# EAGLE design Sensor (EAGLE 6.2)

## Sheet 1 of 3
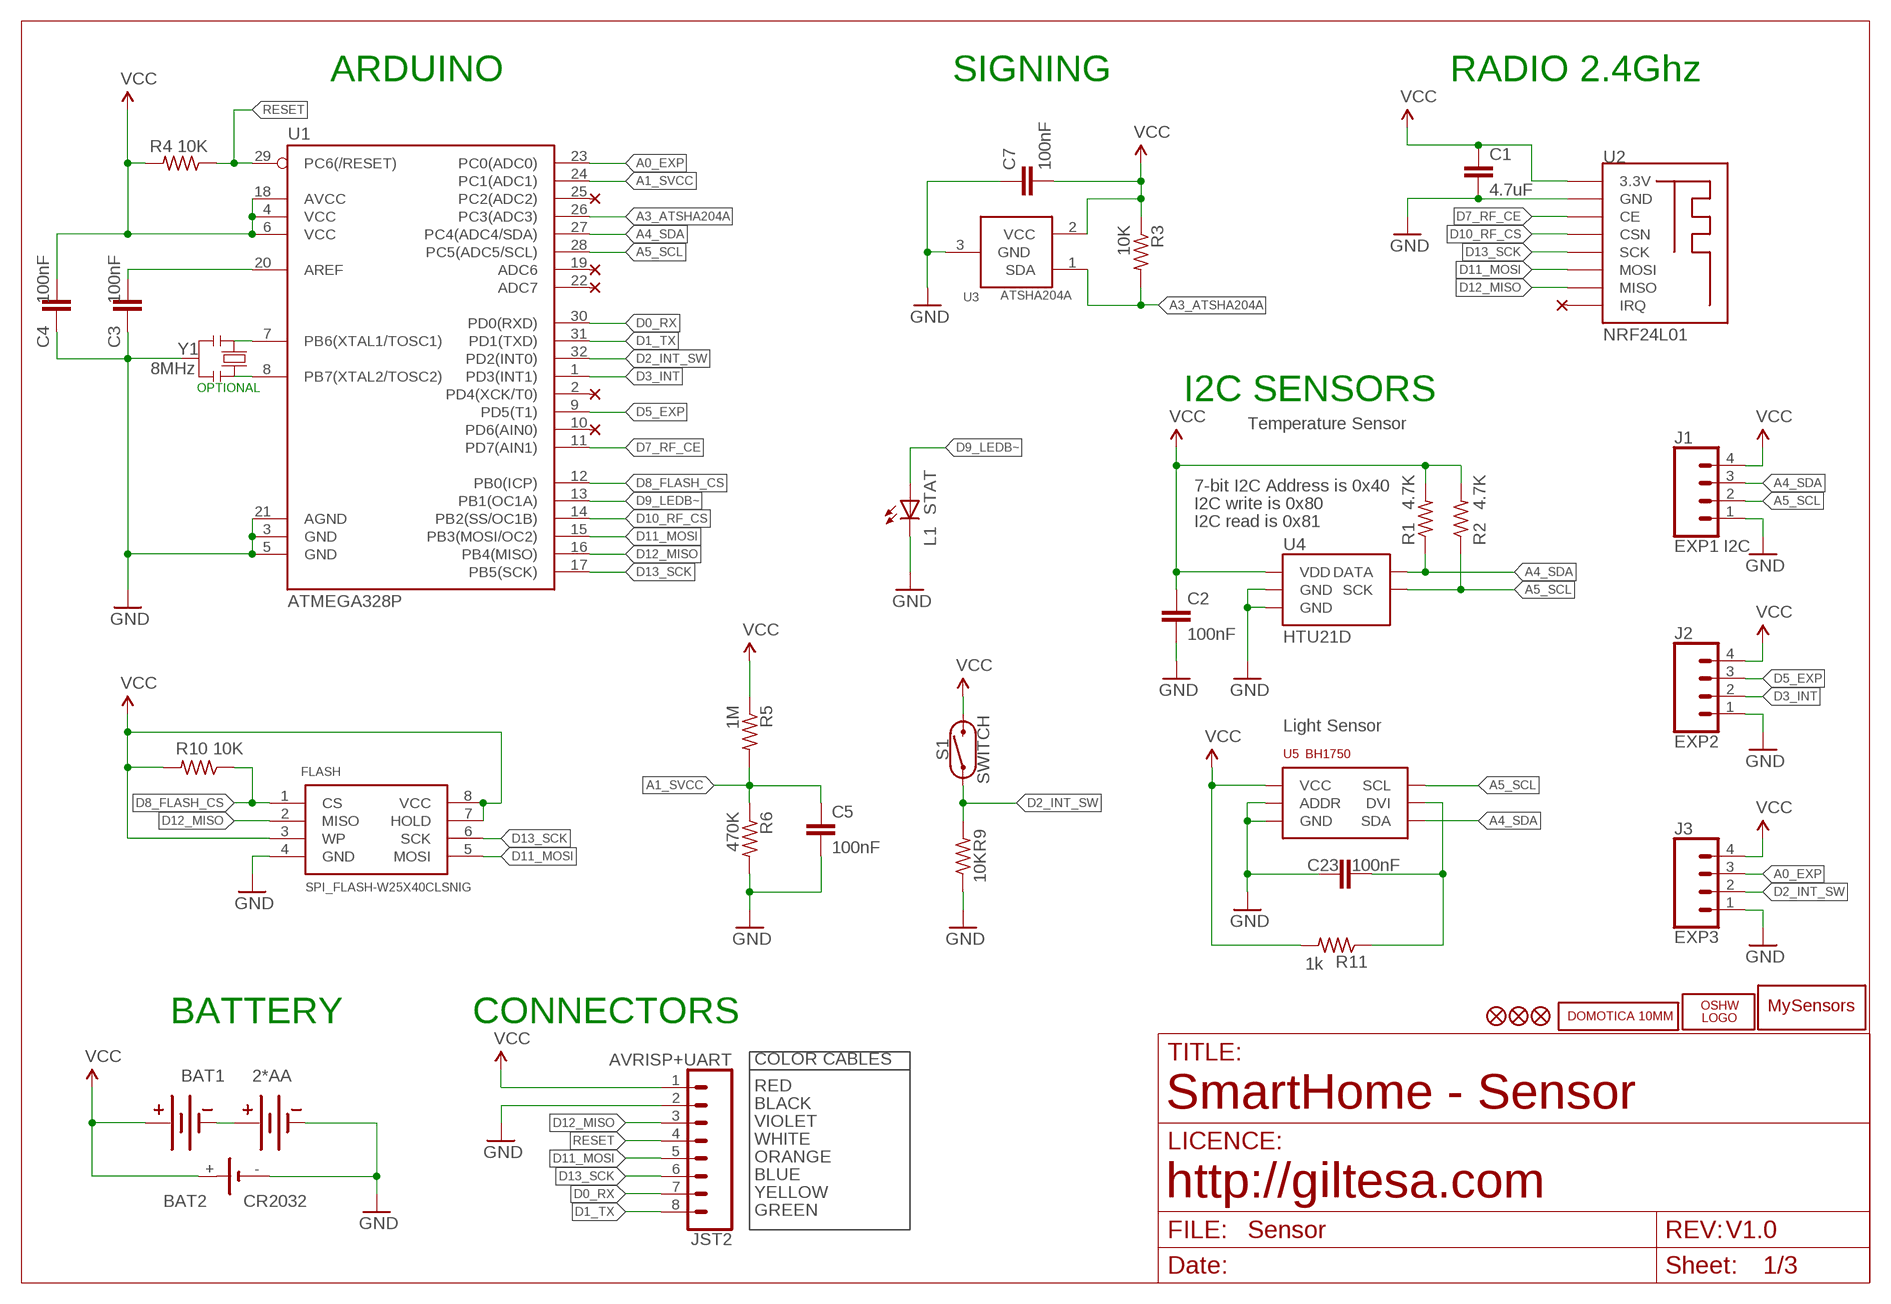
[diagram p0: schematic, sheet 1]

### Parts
BAT1  2*AA  BATTERY_HOLDER_2AA  [BATTERY_HOLDER_2AA]
BAT2  CR2032  CR2032SMD  [CR2032_SMD]
C1  4.7uF  C1206  [C1206]
C2  100nF  C0603  [C0603]
C3  100nF  C0603  [C0603]
C4  100nF  C0603  [C0603]
C5  100nF  C0603  [C0603]
C7  100nF  C0603  [C0603]
C23  100nF  C0603  [C0603]
FLASH  SPI_FLASH-W25X40CLSNIG  SPI_FLASH-X25XXSMD  [SO08]
J1  EXP1 I2C  JST-4-1MM-SMD  [JST-4-1MM-SMD]
J2  EXP2  JST-4-1MM-SMD  [JST-4-1MM-SMD]
J3  EXP3  JST-4-1MM-SMD  [JST-4-1MM-SMD]
JST2  AVRISP+UART  JST-8-1MM-SMD1  [JST-8-1MM-SMD]
L1  STAT  LEDCHIP-LED0805  [CHIP-LED0805]
LOGO1  OSHW_LOGO_FILLX0150-NT  [OSHW_FILLX150_NOTEXT]
R1  4.7K  R0603  [R0603]
R2  4.7K  R0603  [R0603]
R3  10K  R0603  [R0603]
R4  10K  R0603  [R0603]
R5  1M  R0603  [R0603]
R6  470K  R0603  [R0603]
R9  10K  R0603  [R0603]
R10  10K  R0603  [R0603]
R11  1k  R0603  [R0603]
S1  SWITCH  REED_SWITCH-PTH-GLASS  [REED_SWITCH_GLASS]
U1  ATMEGA328P  ATMEGA328P_TQFP  [TQFP32-08]
U2  NRF24L01  NRF24L01_SMD  [NRF24L01_SMD]
U3  ATSHA204A  IC_ATSHA204A_CRYPT  [SOT23-3]
U4  HTU21D  HTU21DSMD  [HTU21D]
U5  BH1750  [BH1750]
U$2  MYSENSORS2  [MYSENSORS_20MM]
U$5  DOMOTICA-10MM  [DOMOTICA-10MM]
U$6  FIDUCIAL1X2  [FIDUCIAL-1X2]
U$7  FIDUCIAL1X2  [FIDUCIAL-1X2]
U$14  FIDUCIAL1X2  [FIDUCIAL-1X2]
Y1  8MHz  RESONATORMU  [RESONATOR]

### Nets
A0_EXP: J3.3 U1.23(PC0(ADC0))
A1_SVCC: C5.1 R5.2 R6.1 U1.24(PC1(ADC1))
A3_ATSHA204A: R3.2 U1.26(PC3(ADC3)) U3.1(SDA)
A4_SDA: J1.3 R1.1 U1.27(PC4(ADC4/SDA)) U4.DATA U5.SDA
A5_SCL: J1.2 R2.1 U1.28(PC5(ADC5/SCL)) U4.SCK U5.SCL
D0_RX: JST2.7 U1.30(PD0(RXD))
D1_TX: JST2.8 U1.31(PD1(TXD))
D2_INT_SW: J3.2 R9.2 S1.P$1 U1.32(PD2(INT0))
D3_INT: J2.2 U1.1(PD3(INT1))
D5_EXP: J2.3 U1.9(PD5(T1))
D7_RF_CE: U1.11(PD7(AIN1)) U2.CE
D8_FLASH_CS: FLASH.1(CS) R10.1 U1.12(PB0(ICP))
D9_LEDB~: L1.A U1.13(PB1(OC1A))
D10_RF_CS: U1.14(PB2(SS/OC1B)) U2.CSN
D11_MOSI: FLASH.5(MOSI) JST2.5 U1.15(PB3(MOSI/OC2)) U2.MOSI
D12_MISO: FLASH.2(MISO) JST2.3 U1.16(PB4(MISO)) U2.MISO
D13_SCK: FLASH.6(SCK) JST2.6 U1.17(PB5(SCK)) U2.SCK
GND: BAT1.GND@1(GND) BAT2.- C1.2 C2.2 C3.1 C4.1 C5.2 C7.1 C23.2 FLASH.4(GND) J1.1 J2.1 J3.1 JST2.2 L1.C R6.2 R9.1 U1.3(GND) U1.5(GND) U1.21(AGND) U2.GND U3.3(GND) U4.7(GND) U4.GND U5.ADDR U5.GND Y1.2
N$1: BAT1.GND@2(GND) BAT1.VCC@1(VCC)
N$19: C23.1 R11.1 U5.DVI
N$29: U1.7(PB6(XTAL1/TOSC1)) Y1.1
N$30: U1.8(PB7(XTAL2/TOSC2)) Y1.3
N$33: C3.2 U1.20(AREF)
RESET: JST2.4 R4.1 U1.29(PC6(/RESET))
VCC: BAT1.VCC@2(VCC) BAT2.+ C1.1 C2.1 C4.2 C7.2 FLASH.3(WP) FLASH.7(HOLD) FLASH.8(VCC) J1.4 J2.4 J3.4 JST2.1 R1.2 R2.2 R3.1 R4.2 R5.1 R10.2 R11.2 S1.P$2 U1.4(VCC) U1.6(VCC) U1.18(AVCC) U2.3.3V U3.2(VCC) U4.VDD U5.VCC
Unconnected: U1.2(PD4(XCK/T0)) U1.10(PD6(AIN0)) U1.19(ADC6) U1.22(ADC7) U1.25(PC2(ADC2)) U2.IRQ

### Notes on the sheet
- ARDUINO | SIGNING | RADIO 2.4Ghz
- OPTIONAL
- I2C SENSORS
- Temperature Sensor
- 7-bit I2C Address is 0x40
- I2C write is 0x80
- I2C read is 0x81
- Light Sensor
- BATTERY | CONNECTORS
- COLOR CABLES
- RED
- BLACK | SmartHome - Sensor
- VIOLET
- WHITE
- ORANGE
- BLUE
- YELLOW | http://giltesa.com
- GREEN
- V1.0

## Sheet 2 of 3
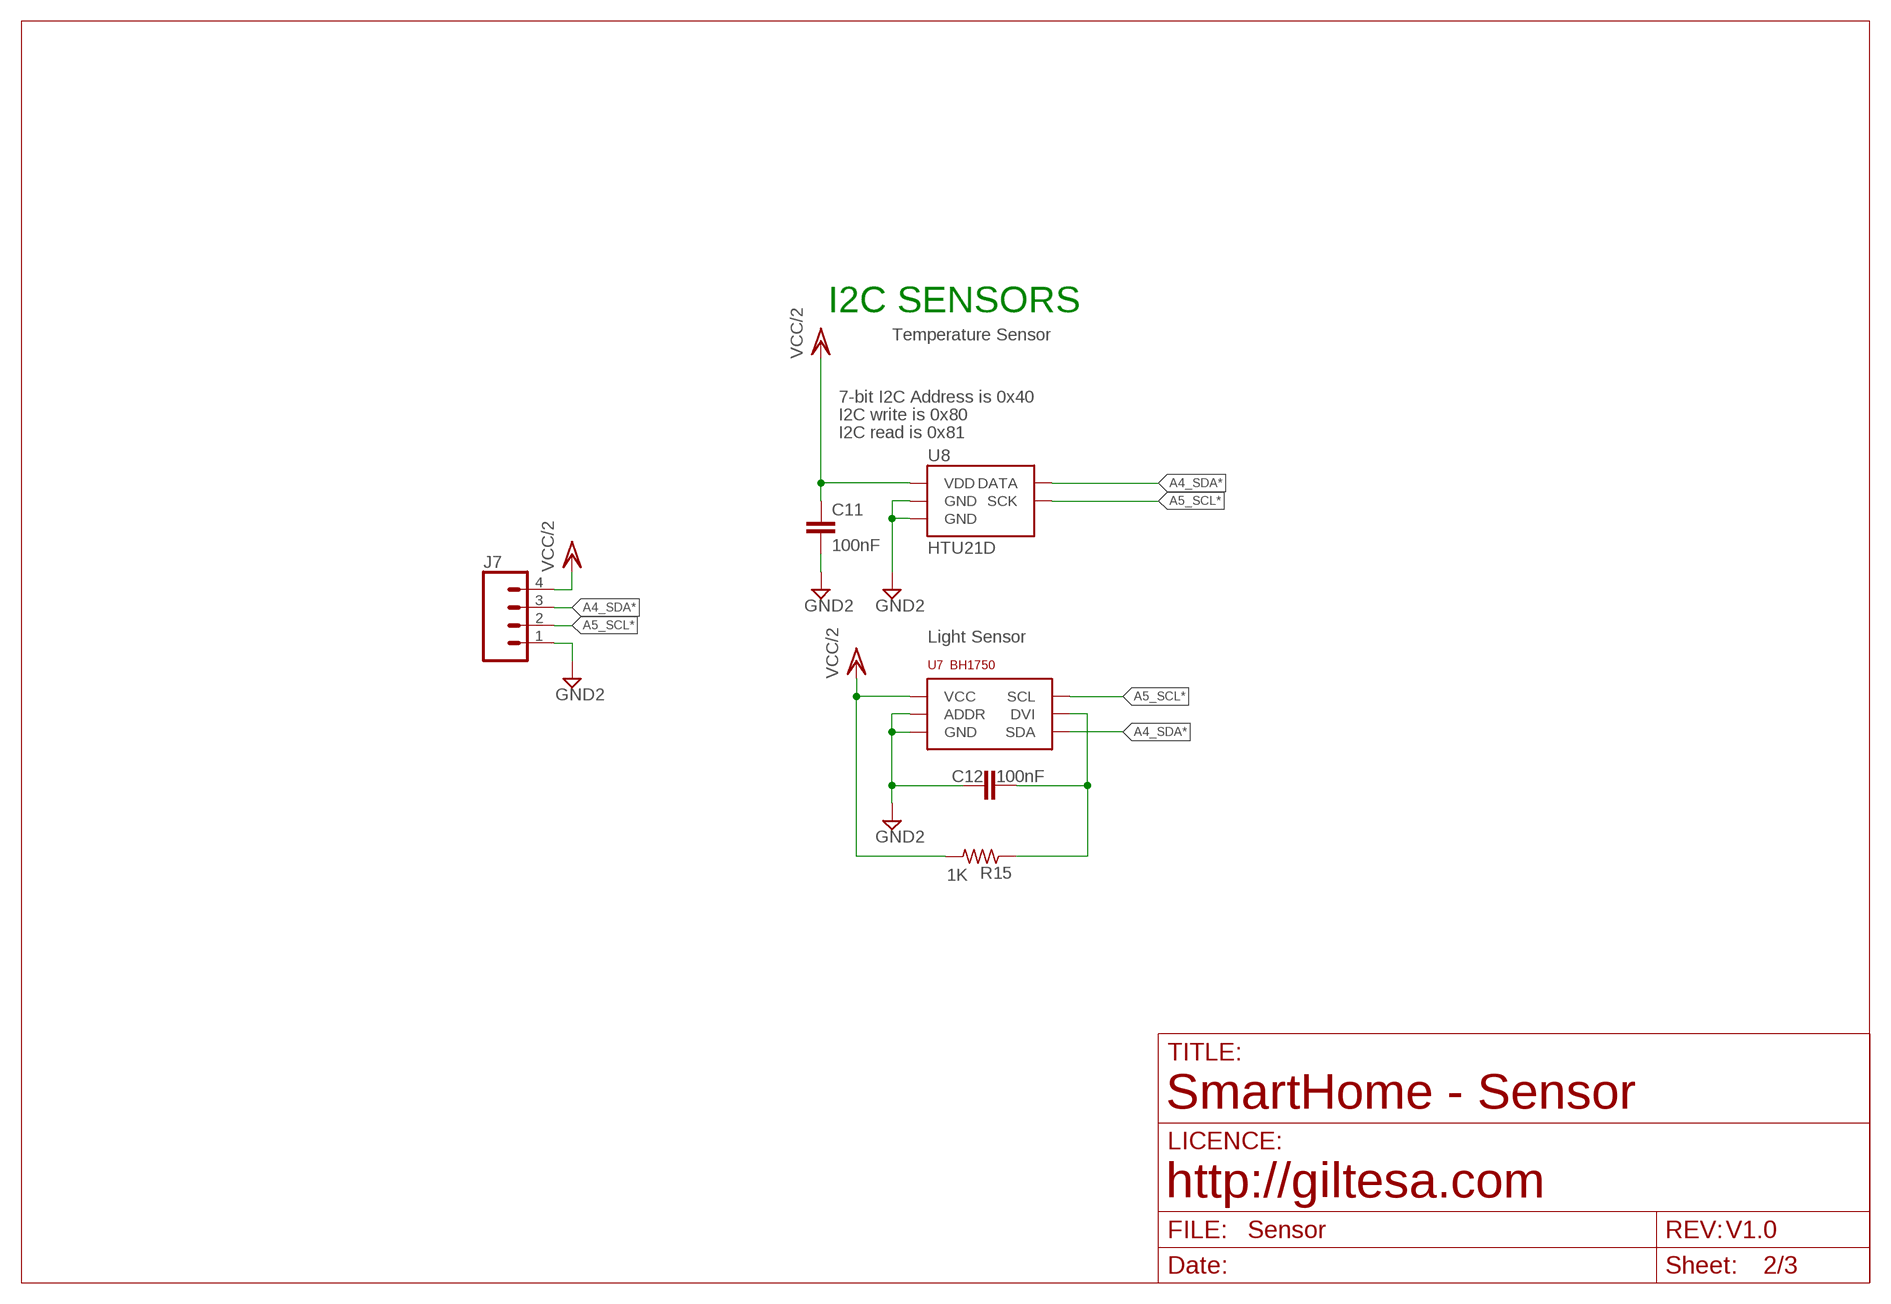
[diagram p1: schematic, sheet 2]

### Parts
C11  100nF  C0603  [C0603]
C12  100nF  C0603  [C0603]
J7  CONN_041X04_NO_SILK  [1X04_NO_SILK]
R15  1K  R0603  [R0603]
U7  BH1750  [BH1750]
U8  HTU21D  HTU21DSMD  [HTU21D]

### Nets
A4_SDA*: J7.3 U7.SDA U8.DATA
A5_SCL*: J7.2 U7.SCL U8.SCK
GND2: C11.2 C12.2 J7.1 U7.ADDR U7.GND U8.7(GND) U8.GND
N$5: C12.1 R15.1 U7.DVI
VCC/2: C11.1 J7.4 R15.2 U7.VCC U8.VDD

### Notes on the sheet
- I2C SENSORS
- Temperature Sensor
- 7-bit I2C Address is 0x40
- I2C write is 0x80
- I2C read is 0x81
- Light Sensor
- SmartHome - Sensor
- http://giltesa.com
- V1.0

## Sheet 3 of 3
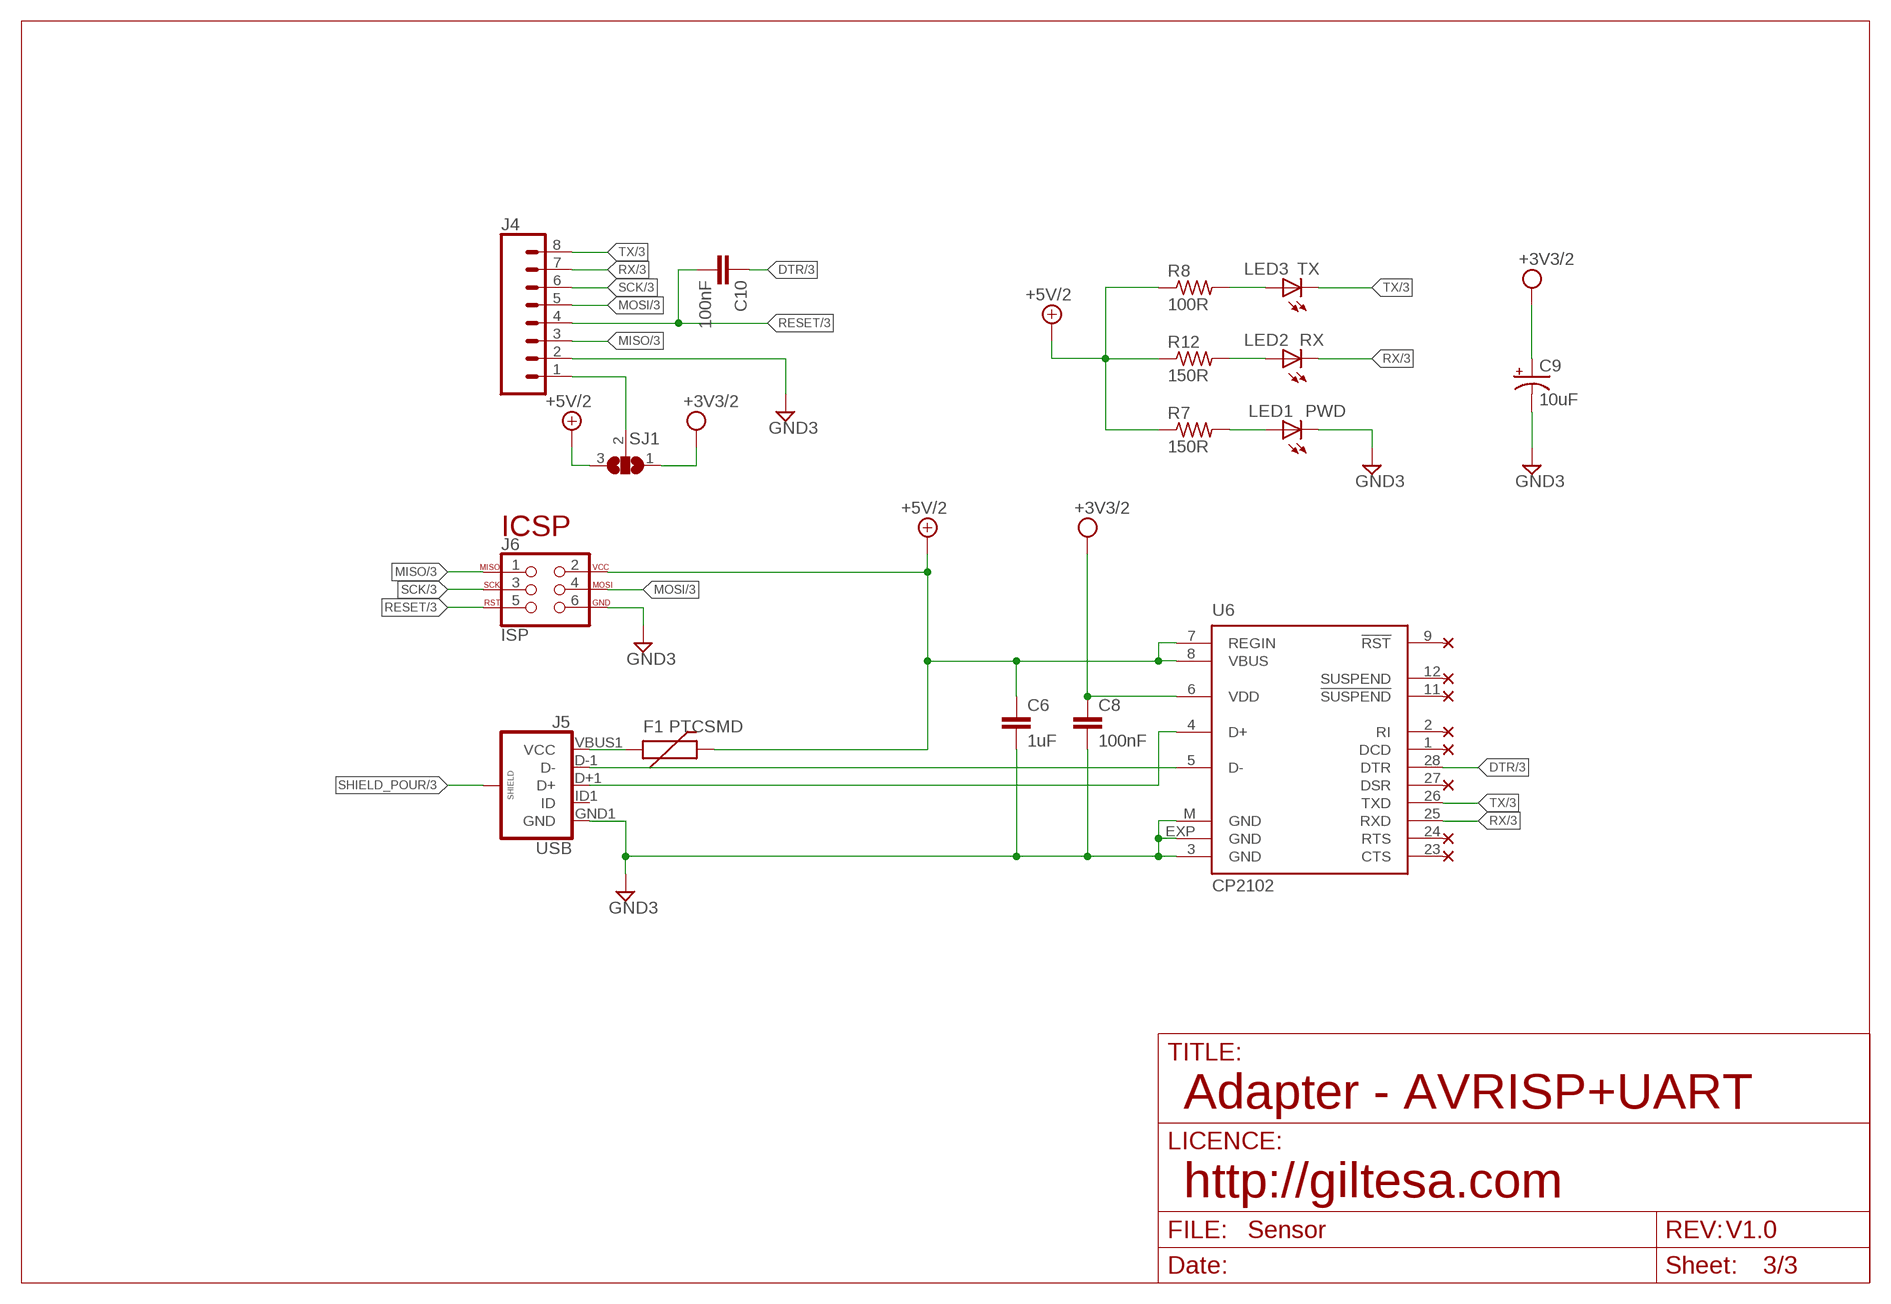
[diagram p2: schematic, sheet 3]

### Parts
C6  1uF  C0603  [C0603]
C8  100nF  C0603  [C0603]
C9  10uF  10UF-16V-10%(TANT)  [EIA3216]
C10  100nF  C0603  [C0603]
F1  PTCSMD  [PTC-1206]
J4  JST-8-1MM-SMD2  [1X08_SMD_2MM]
J5  USB  USB_MICROB_PLUGCONN-11752  [USB-B-MICRO-SMD_V03]
J6  ISP  AVR_SPI_PROG_3X22  [2X03_SMD_REV]
LED1  PWD  LEDCHIP-LED0805  [CHIP-LED0805]
LED2  RX  LEDCHIP-LED0805  [CHIP-LED0805]
LED3  TX  LEDCHIP-LED0805  [CHIP-LED0805]
R7  150R  R0603  [R0603]
R8  100R  R0603  [R0603]
R12  150R  R0603  [R0603]
SJ1  SOLDERJUMPER_2WAYS  [SJ_3]
U6  CP2102  CP210X_USB_UART  [MLP28]

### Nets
+3V3/3: C8.1 C9.A(+) SJ1.1 U6.6(VDD) ; supply symbol labelled +3V3/2
+5V/3: C6.1 F1.2 J6.2 R7.1 R8.1 R12.1 SJ1.3 U6.7(REGIN) U6.8(VBUS) ; supply symbol labelled +5V/2
D+: J5.D+1(D+) U6.4(D+)
D-: J5.D-1(D-) U6.5(D-)
DTR/3: C10.1 U6.28(DTR)
GND3: C6.2 C8.2 C9.C(-) J4.2 J5.GND1(GND) J6.6 LED1.C U6.3(GND) U6.EXP(GND) U6.M(GND)
MISO/3: J4.3 J6.1
MOSI/3: J4.5 J6.4
N$2: LED1.A R7.2
N$3: F1.1 J5.VBUS1(VCC)
N$4: J4.1 SJ1.2
N$6: LED3.A R8.2
N$7: LED2.A R12.2
RESET/3: C10.2 J4.4 J6.5
RX/3: J4.7 LED2.C U6.25(RXD)
SCK/3: J4.6 J6.3
SHIELD_POUR/3: J5.SHIELD1(SHIELD) J5.SHIELD2(SHIELD) J5.SHIELD3(SHIELD)
TX/3: J4.8 LED3.C U6.26(TXD)
Unconnected: J5.ID1(ID) U6.1(DCD) U6.2(RI) U6.9(!RST) U6.11(!SUSPEND) U6.12(SUSPEND) U6.23(CTS) U6.24(RTS) U6.27(DSR)

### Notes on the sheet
- ICSP
- Adapter - AVRISP+UART
- http://giltesa.com
- V1.0

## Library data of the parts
BAT1 = ,giltesa:BATTERY_HOLDER_2AA
BAT2 = ,giltesa:CR2032
C1 = ,giltesa:C1206
C2-C8 C10-C12 C23 = ,giltesa:C0603
C9 = SparkFun-Capacitors:10UF-16V-10%(TANT): CAP-00811; PROD_ID: CAP-00811
F1 = SparkFun:PTC: Resettable Fuse PTC
FLASH = SparkFun-DigitalIC:SPI_FLASH-X25XX: 8pin SPI Flash series x25xx. Works with devices like W25X32 and BR25L32
J1-J3 = ,giltesa:JST-4-1MM-SMD
J4 JST2 = ,giltesa:JST-8-1MM-SMD
J5 = SparkFun-Connectors:USB_MICROB_PLUG: USB Micro-B connectors Some male, some female. Watch your step!; PROD_ID: CONN-11752
J6 = ,giltesa:AVR_SPI_PROG_3X2
J7 = SparkFun-Connectors:CONN_04: Multi connection point. Often used as Generic Header-pin footprint for 0.1 inch spaced/style header connections On any of the 0.1 inch spaced packages, you can populate with these: Break Away Headers - Straight (PRT-00116) Break Away Male Headers - Right Angle (PRT-00553) Female Headers (PRT-00115)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; PROD_ID: CONN-09696
L1 LED1-LED3 = led:LED: LED
LOGO1 = ohw-logo:OSHW_LOGO_FILL
R1-R12 R15 = ,giltesa:R0603
S1 = SparkFun-Switches:REED_SWITCH: Reed Switch; PROD_ID: SWCH-09282; SF_SKU: COM-08642
SJ1 = SparkFun:SOLDERJUMPER_2WAY: Solder Jumper 2 way solder jumper
U1 = SparkFun-DigitalIC:ATMEGA328P_TQFP; PROD_ID: IC-09069; VALUE: ATMEGA328P_TQFP
U2 = ,giltesa:NRF24L01_SMD
U3 = TD-MySensors:IC_ATSHA204A_CRYPT
U4 U8 = SparkFun-Sensors:HTU21D
U5 U7 = ,giltesa:BH1750
U6 = SparkFun:CP210X_USB_UART: Single-Chip USB to UART Bridge Source: www.silabs.com .. CP2101.pdf / cp2102.pdf. Spark Fun Electronics SKU : COM-00310
U$2 = ,giltesa_logos:MYSENSORS
U$5 = ,giltesa_logos:DOMOTICA-10MM
U$6 U$7 U$14 = SparkFun:FIDUCIAL: Fiducial Alignment Points
Y1 = MySMD2:RESONATOR

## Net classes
2 gnd: width 0.305 mm, drill 0.406 mm, clearance 0.203 mm
3 usbvcc: width 0.203 mm, drill 0.406 mm, clearance 0.203 mm
4 USBpair: width 0.254 mm, drill 0.406 mm, clearance 0.61 mm

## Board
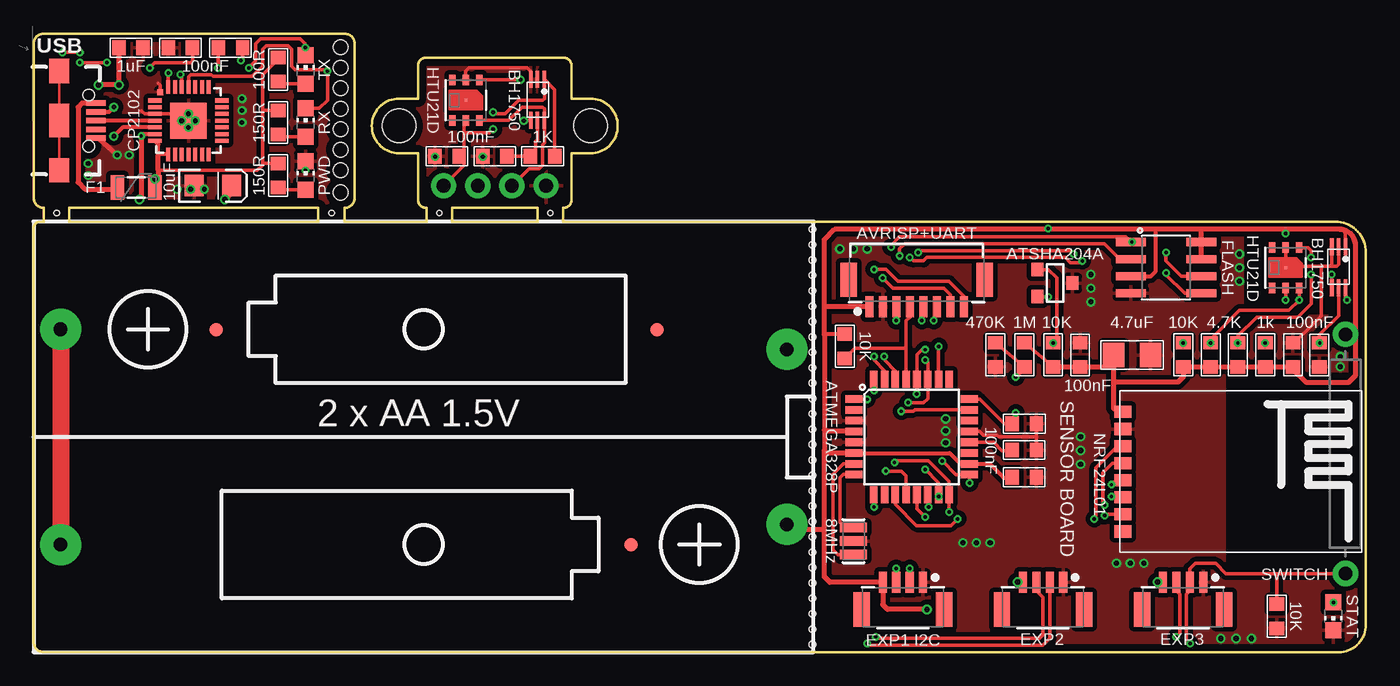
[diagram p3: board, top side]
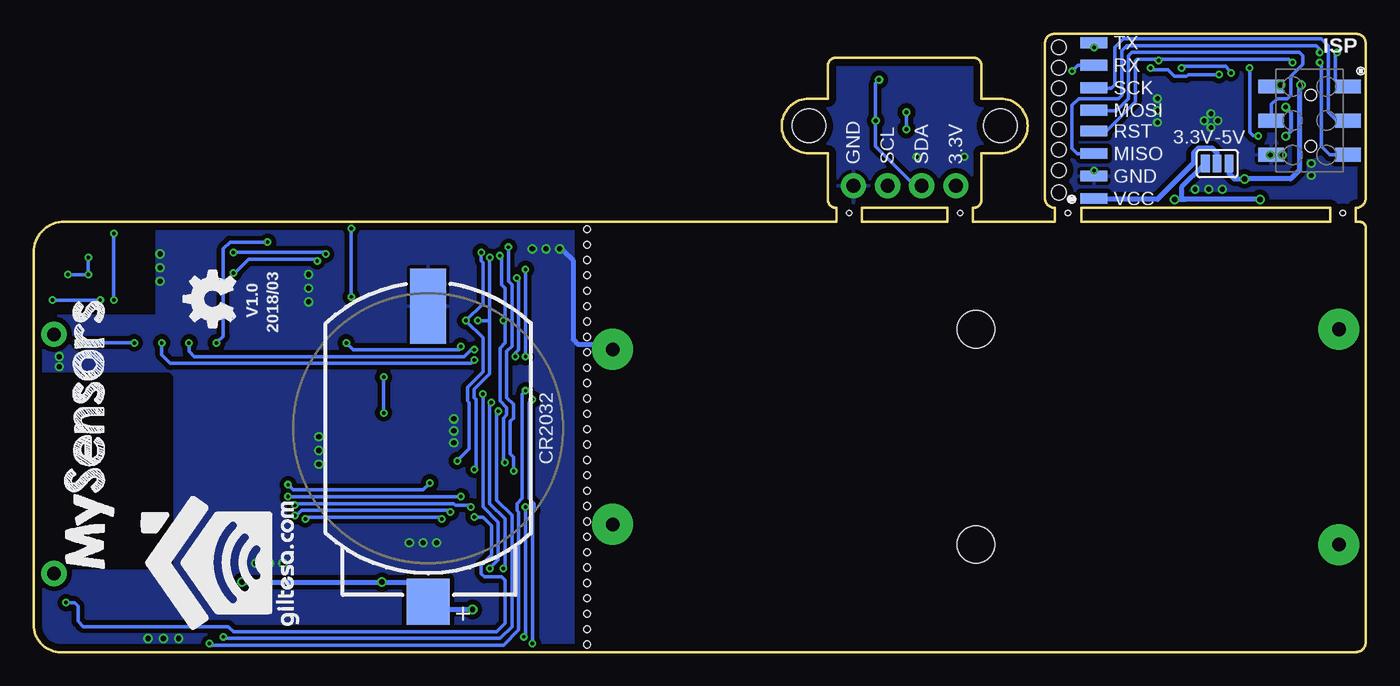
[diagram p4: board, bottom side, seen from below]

Size 99.06 x 45.97 mm. Coordinates in mm from the lower left corner, seen from the top.
Outline: 2.66,33.03 21.14,33.03 21.14,32 2.66,32 2.66,33.03
Outline: 0.76,0 97.03,0 arc90 99.06,2.03 99.06,29.72 arc90 96.77,32 39.37,32 39.37,33.02 arc90 40.01,33.66 40.01,37.08 41.4,37.08 arc90 43.43,39.12 arc90 41.4,41.15 40.01,41.15 40.01,43.56 arc90 39.37,44.2 29.21,44.2 arc90 28.57,43.56 28.57,41.15 27.18,41.15 arc90 25.15,39.12 arc90 27.18,37.08 28.57,37.08 28.57,33.66 arc90 29.21,33.02 29.21,32 23.11,32 23.11,33.02 arc90 23.88,33.78 23.88,45.21 arc90 23.11,45.97 0.76,45.97 arc90 0,45.21 0,33.78 arc90 0.76,33.02 0.76,32 0.51,32 arc90 0,31.5 0,0.76 arc90 0.76,0
Outline: 37.47,32 31.11,32 31.11,33.02 37.47,33.02 37.47,32
Copper layers (1*16): Top 0.035mm / dielectric 1.6mm / Bottom 0.035mm
Design rules: minimum track width 6mil, minimum drill 12mil, track to track 6mil, track to pad 6mil, pad to pad 6mil, via to via 8mil, smd to smd 0mil, copper to edge 20mil, drill to drill 10mil, minimum pad ring 6mil, minimum via ring 6mil, stop-mask expansion 0mil, vias tented up to drill 100mil, thermal gap 10mil
Holes 0.51 mm at 57.91,0.57 57.91,1.71 57.91,2.86 57.91,4 57.91,5.14 57.91,6.29 57.91,7.43 57.91,8.57 57.91,9.72 57.91,10.86 57.91,12 57.91,13.14 57.91,14.29 57.91,15.43 57.91,16.57 57.91,17.72 57.91,18.86 57.91,20 57.91,21.15 57.91,22.29 57.91,23.43 57.91,24.57 57.91,25.72 57.91,26.86 57.91,28 57.91,29.15 57.91,30.29 57.91,31.43
Holes 1.1 mm at 22.82,35.82 22.82,37.35 22.82,38.87 22.82,40.39 22.82,41.92 22.82,43.44 22.82,44.97 22.82,34.17
Holes 0.4 mm at 22.16,32.64 1.71,32.64 30.16,32.64 38.41,32.64
Holes 2.79 mm at 29.01,24 29.01,8
Holes 2.5 mm at 27.18,39.12 41.4,39.12
tRestrict: 4 lines
bRestrict: 4 lines

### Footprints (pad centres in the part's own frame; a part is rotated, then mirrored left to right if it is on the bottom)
BATTERY_HOLDER_2AA = drill 1.016 pad 3.048: GND@1 56,22.5; GND@2 2,8; VCC@1 2,24; VCC@2 56,9.5
CR2032_SMD = smd 3.429 x 3.175: + 12.896,0 | smd 5.588 x 2.667: - -9.075,0
C1206 = smd 1.6 x 1.8: 1 -1.362,-0.013; 2 1.387,-0.013
C0603 = smd 1 x 1.1: 1 -0.901,-0.038; 2 0.901,-0.038
EIA3216 = smd 1.4 x 1.6: A 1.4,0; C -1.4,0
PTC-1206 = smd 1 x 1.8: 1 -1.4,0; 2 1.4,0
SO08 = smd 0.61 x 2.21: 1 -1.905,-2.616; 2 -0.635,-2.616; 3 0.635,-2.616; 4 1.905,-2.616; 5 1.905,2.616; 6 0.635,2.616; 7 -0.635,2.616; 8 -1.905,2.616
JST-4-1MM-SMD = smd 0.6 x 1.55: 1 -1.493,-2.017; 2 -0.493,-2.017; 3 0.507,-2.017; 4 1.507,-2.017 | smd 1.219 x 2.54: P$5 3.06,0; P$6 -3.047,0
1X08_SMD_2MM = smd 2 x 0.8: 1 0,-5.792; 2 0,-4.119; 3 0,-2.446; 4 0,-0.773; 5 0,0.773; 6 0,2.446; 7 0,4.119; 8 0,5.792
USB-B-MICRO-SMD_V03 = smd 1.45 x 0.4: D+1 2.725,0; D-1 2.725,0.65; GND1 2.725,-1.3; ID1 2.725,-0.65; VBUS1 2.725,1.3 | smd 1.5 x 1.8: SHIELD1 0,3.685; SHIELD2 0,-3.685 | smd 1.5 x 2.5: SHIELD3 0,0 | hole 0.85: 2.2,1.9; 2.2,-1.9
2X03_SMD_REV = smd 1.9 x 1.02 bottom: 1 -2.85,2.54; 2 2.85,2.54; 3 -2.85,0; 4 2.85,0; 5 -2.85,-2.54; 6 2.85,-2.54
1X04_NO_SILK = drill 1.016 pad 1.88: 1 0,0; 2 2.54,0; 3 5.08,0; 4 7.62,0
JST-8-1MM-SMD = smd 0.6 x 1.55: 1 -3.5,-2.017; 2 -2.5,-2.017; 3 -1.5,-2.017; 4 -0.5,-2.017; 5 0.5,-2.017; 6 1.5,-2.017; 7 2.5,-2.017; 8 3.5,-2.017 | smd 1.219 x 2.54: NC1 -5.054,0; NC2 5.054,0
CHIP-LED0805 = smd 1.2 x 1.2: A 0,-1.05; C 0,1.05
R0603 = smd 1 x 1.1: 1 -0.901,0.013; 2 0.901,0.013
REED_SWITCH_GLASS = drill 1.016 pad 1.88: P$1 -8.89,0; P$2 8.89,0
SJ_3 = smd 0.635 x 1.27: 1 -0.889,0; 2 0,0; 3 0.889,0
TQFP32-08 = smd 1.27 x 0.559: 1 -4.293,2.8; 2 -4.293,2; 3 -4.293,1.2; 4 -4.293,0.4; 5 -4.293,-0.4; 6 -4.293,-1.2; 7 -4.293,-2; 8 -4.293,-2.8; 17 4.293,-2.8; 18 4.293,-2; 19 4.293,-1.2; 20 4.293,-0.4; 21 4.293,0.4; 22 4.293,1.2; 23 4.293,2; 24 4.293,2.8 | smd 0.559 x 1.27: 9 -2.8,-4.293; 10 -2,-4.293; 11 -1.2,-4.293; 12 -0.4,-4.293; 13 0.4,-4.293; 14 1.2,-4.293; 15 2,-4.293; 16 2.8,-4.293; 25 2.8,4.293; 26 2,4.293; 27 1.2,4.293; 28 0.4,4.293; 29 -0.4,4.293; 30 -1.2,4.293; 31 -2,4.293; 32 -2.8,4.293
NRF24L01_SMD = smd 0.9 x 1.27: 3.3V 1.575,0.203; CE 4.115,0.203; CSN 5.385,0.203; GND 2.845,0.203; IRQ 10.465,0.203; MISO 9.195,0.203; MOSI 7.925,0.203; SCK 6.655,0.203
SOT23-3 = smd 1 x 0.9: 1 -1,-1.3; 2 1,-1.3; 3 0,1.3
HTU21D = smd 0.2 x 0.2: 7 0,0 | smd 0.8 x 0.5: DATA 1.5,-1; GND 1.5,0; NC@1 -1.5,1; NC@6 1.5,1; SCK -1.5,-1; VDD -1.5,0
BH1750 = smd 1.27 x 0.27: ADDR -1.549,0; DVI 1.499,0; GND -1.549,-0.508; SCL 1.499,0.508; SDA 1.499,-0.508; VCC -1.549,0.508
MLP28 = smd 1 x 0.3: 1 -2.5,1.5; 2 -2.5,1; 3 -2.5,0.5; 4 -2.5,0; 5 -2.5,-0.5; 6 -2.5,-1; 7 -2.5,-1.5; 15 2.5,-1.5; 16 2.5,-1; 17 2.5,-0.5; 18 2.5,0; 19 2.5,0.5; 20 2.5,1; 21 2.5,1.5 | smd 0.3 x 1: 8 -1.5,-2.5; 9 -1,-2.5; 10 -0.5,-2.5; 11 0,-2.5; 12 0.5,-2.5; 13 1,-2.5; 14 1.5,-2.5; 22 1.5,2.5; 23 1,2.5; 24 0.5,2.5; 25 0,2.5; 26 -0.5,2.5; 27 -1,2.5; 28 -1.5,2.5 | smd 2.7 x 2.7: EXP 0,0 | smd 0.435 x 0.435: M -2.103,2.103
FIDUCIAL-1X2 = smd 1 x 1: 1 0,0
RESONATOR = smd 0.7 x 2: 1 -1,0; 2 0,0; 3 1,0

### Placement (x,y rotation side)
BAT1  0,0 0 top
BAT2  69.72,16.64 270 bottom
C1  81.66,22.1 0 top
C2  93.6,22.1 90 top
C3  73.66,14.99 180 top
C4  73.66,12.95 180 top
C5  73.66,17.02 0 top
C6  7.24,44.96 0 top
C7  77.85,22.1 270 top
C8  10.92,44.88 180 top
C9  13.34,34.67 0 top
C10  14.64,44.96 0 top
C11  30.73,36.83 180 top
C12  34.29,36.83 180 top
C23  95.63,22.1 270 top
F1  7.62,34.54 0 top
FLASH  84.2,28.57 270 top
J1  64.64,3.17 180 top
J2  75.06,3.17 180 top
J3  85.47,3.17 180 top
J4  20.23,39.51 0 bottom
J5  1.91,39.51 0 top
J6  4.19,39.51 0 top
J7  38.1,34.67 180 top
JST2  65.66,27.69 0 top
L1  96.65,2.67 180 top
LED1  20.23,35.43 0 top
LED2  20.23,39.37 0 top
LED3  20.23,43.31 0 top
LOGO1  84.07,24.13 90 bottom
R1  89.53,22.1 270 top
R2  87.5,22.1 270 top
R3  75.82,22.1 90 top
R4  60.33,22.73 90 top
R5  73.66,22.1 270 top
R6  71.5,22.1 270 top
R7  18.16,35.43 270 top
R8  18.16,43.31 270 top
R9  92.46,2.67 90 top
R10  85.47,22.1 270 top
R11  91.57,22.1 270 top
R12  18.16,39.37 270 top
R15  37.85,36.86 0 top
S1  97.54,14.73 90 top
SJ1  11.05,36.32 0 bottom
U1  65.28,16 0 top
U2  80.77,19.43 270 top
U3  75.95,27.43 270 top
U4  93.09,28.57 90 top
U5  97.03,28.57 270 top
U6  11.52,39.51 0 top
U7  37.47,41.02 270 top
U8  32.13,41.02 90 top
U$2  93.09,6.22 90 bottom
U$5  79.25,1.65 90 bottom
U$6  46.35,23.98 0 top
U$7  13.59,23.98 0 top
U$14  44.42,8 0 top
Y1  60.96,8.26 90 top

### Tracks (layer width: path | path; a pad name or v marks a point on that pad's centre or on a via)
+3V3/3  (via drill 0.25, 0.41)
  Top 0.254: C8.1 11.82,43.95 11.68,43.81 9.02,43.81 v8.64,43.43
  Top 0.305: U6.6 8.41,38.51 8.15,38.51 v8,38.35
  Top 0.356: C9.A 14.73,34.16 v14.22,33.66 | v8,38.35 8,33.78 v7.87,33.66
  Bottom 0.254: v8.64,43.43 8.64,38.63 8.38,38.38 7.9,38.38 v8,38.35
  Bottom 0.356: v7.87,33.66 13.46,33.66 13.59,33.66 | SJ1.1 11.94,36.2 12.06,36.2 13.72,34.54 13.72,33.78 13.59,33.66 | v14.22,33.66 13.59,33.66
+5V/3  (via drill 0.41)
  Top 0.254: R8.1 18.17,44.08 17.02,42.93 17.02,40.39 | 17.02,40.39 17.02,36.32 | 17.02,36.32 17.02,36.2 16.64,35.81 9.27,35.81 | R12.1 17.13,40.27 17.02,40.39 | R7.1 17.03,36.33 17.02,36.32
  Top 0.305: 9.27,36.96 9.27,37.08 | 9.27,37.08 9.27,37.75 U6.7 | U6.8 9.35,37.01 9.27,37.08
  Top 0.356: 9.27,36.96 9.27,35.81 9.27,34.8 v9.02,35.18 F1.2 | C6.1 6.34,42.3 v6.35,42.16 v4.83,42.16
  Bottom 0.356: 7.74,42.05 J6.2 6.92,42.16 v6.35,42.16 | v4.83,42.16 4.95,42.04 4.95,35.81 5.59,35.18 v9.02,35.18 9.78,35.18 10.16,35.56 SJ1.3
A0_EXP  (via drill 0.25)
  Top 0.254: v64.52,17.91 65.41,17.91 65.53,18.03 69.54,18.03 U1.23 | J3.3 84.96,4.57 85.22,4.32 85.22,1.4 v84.96,1.14
  Bottom 0.254: v84.96,1.14 84.84,1.02 64.39,1.02 63.5,1.91 63.5,10.16 64.64,11.3 64.64,17.78 v64.52,17.91
A1_SVCC  (via drill 0.25)
  Top 0.254: R6.1 R5.2 73.67,21.09 v73.03,20.45 | U1.24 70.35,18.8 72.17,16.98 C5.1 | C5.1 72.76,17.01 | v73.03,17.78 73.03,17.25 C5.1
  Bottom 0.254: v73.03,20.45 v73.03,17.78
A3_ATSHA204A  (via drill 0.25)
  Top 0.254: U3.1 75.45,28.43 76.07,27.81 76.07,23.39 R3.2 v75.82,22.99 | U1.26 67.28,22.7 v67.31,22.73
  Bottom 0.254: v75.82,22.99 75.31,22.48 67.44,22.48 67.31,22.61 v67.31,22.73
A4_SDA  (via drill 0.25)
  Top 0.254: R1.1 89.55,23.51 | 89.55,23.51 90.93,24.89 93.98,24.89 95,25.91 v95,28.07 | v96.52,28.07 U5.SDA | U4.DATA 94.77,30.07 95,29.84 v95,29.34 | v65.02,18.54 66.17,18.54 66.48,18.85 U1.27 66.48,21.53 v66.29,21.72 | v64.14,6.22 J1.3 | v89.53,22.99 89.53,23.5 89.55,23.51
  Bottom 0.254: v96.52,28.07 v95,28.07 v95,29.34 | v64.14,6.22 64.01,6.35 64.01,9.91 65.15,11.05 65.15,18.41 v65.02,18.54 | v89.53,22.99 89.53,22.1 88.9,21.46 66.55,21.46 v66.29,21.72
A4_SDA*  (via drill 0.3)
  Top 0.254: U7.SDA 36.47,39.52 v36.45,39.5 | v36.2,42.55 33.16,42.55 U8.DATA
  Bottom 0.254: v36.2,42.55 36.45,42.29 v36.45,39.5 36.45,37.59 33.53,34.67 J7.3
A5_SCL  (via drill 0.25)
  Top 0.254: U5.SCL 97.54,26.29 v97.66,26.16 | U4.SCK 94.11,27.06 v94.11,26.16 93.34,25.4 89.66,25.4 87.52,23.25 R2.1 v87.5,22.99 | v65.66,19.18 65.68,19.2 U1.28 65.68,22.12 66.04,22.48 v66.29,22.48 | v65.15,6.22 65.15,5.21 J1.2
  Bottom 0.254: v97.66,26.16 v94.11,26.16 | v65.15,6.22 64.52,6.86 64.52,9.65 65.66,10.79 v65.66,19.18 | v87.5,22.99 87.5,22.35 87.12,21.97 67.06,21.97 66.55,22.48 v66.29,22.48
A5_SCL*
  Top 0.254: U8.SCK 35.33,39.52 36.32,40.51 37.85,40.51 37.97,40.39 U7.SCL 37.97,37.85 37.85,37.72 37.85,36.2 37.59,35.94 36.83,35.94 J7.2
D0_RX  (via drill 0.25)
  Top 0.254: v63.25,21.97 63.25,21.72 64.08,20.89 U1.30 | v63.12,27.81 63.88,27.05 67.69,27.05 68.16,26.58 JST2.7
  Bottom 0.254: v63.25,21.97 63.25,22.23 62.99,22.48 62.99,27.81 v63.12,27.81
D1_TX  (via drill 0.25)
  Top 0.254: v62.48,21.97 62.48,21.72 63.28,20.92 U1.31 | v62.48,28.45 63.37,28.45 64.26,27.56 68.07,27.56 69.16,26.47 JST2.8
  Bottom 0.254: v62.48,21.97 v62.48,28.45
D2_INT_SW  (via drill 0.25)
  Top 0.254: S1.P$1 92.46,5.84 | 92.46,5.84 88.65,5.84 87.88,6.6 86.36,6.6 85.96,6.21 J3.2 85.98,5.18 85.98,4.57 85.72,4.32 85.72,0.89 v85.98,0.64 | R9.2 92.44,5.83 92.46,5.84 | v62.48,19.43 U1.32
  Bottom 0.254: 62.61,19.3 v62.48,19.43 62.74,19.18 62.74,11.43 63.12,11.05 63.12,10.54 62.99,10.41 62.99,1.65 64.14,0.51 85.85,0.51 v85.98,0.64
D3_INT  (via drill 0.25)
  Top 0.254: U1.1 v61.98,18.8 | v61.98,0.64 62.1,0.51 75.06,0.51 75.56,1.02 75.56,5.18 J2.2
  Bottom 0.254: 62.1,18.67 v61.98,18.8 62.23,18.54 62.23,11.43 61.85,11.05 61.85,10.54 61.98,10.41 v61.98,0.64
D5_EXP  (via drill 0.25)
  Top 0.254: v62.48,10.79 U1.9 | v62.61,1.14 62.74,1.02 74.8,1.02 75.06,1.27 75.06,4.06 74.55,4.57 J2.3
  Bottom 0.254: v62.48,10.79 62.48,1.27 v62.61,1.14
D7_RF_CE  (via drill 0.25)
  Top 0.254: U1.11 64.08,10.98 65.66,9.4 68.2,9.4 v68.71,9.91 | U2.CE 80.59,15.32 78.99,13.72 78.99,10.03 v78.87,9.91
  Bottom 0.254: v68.71,9.91 68.83,10.03 78.74,10.03 v78.87,9.91
D8_FLASH_CS  (via drill 0.25)
  Top 0.254: U1.12 64.88,13.1 64.52,13.46 v63.37,13.46 | v63.75,30.1 63.75,30.23 64.39,30.86 81.2,30.86 FLASH.1 v81.66,30.48 | v85.47,22.99 R10.1
  Bottom 0.254: v63.37,13.46 63.37,14.48 63.63,14.73 63.63,17.14 63.37,17.4 63.37,18.41 63.88,18.92 63.88,22.35 63.5,22.73 63.5,27.3 63.75,27.56 v63.75,30.1 | v85.47,22.99 84.96,23.5 84.96,29.97 84.45,30.48 v81.66,30.48
D9_LEDB~  (via drill 0.25)
  Top 0.254: U1.13 65.68,10.65 v66.29,10.03 | v96.65,3.68 96.61,3.68 L1.A
  Bottom 0.254: v96.65,3.68 96.01,3.68 95.76,3.43 95.76,2.29 95.38,1.91 84.58,1.91 84.2,1.52 64.64,1.52 64.01,2.16 64.01,5.33 64.26,5.59 65.53,5.59 65.79,5.84 65.79,6.48 65.02,7.24 65.02,9.4 65.66,10.03 v66.29,10.03
D10_RF_CS  (via drill 0.25)
  Top 0.254: U2.CSN 80.21,14.05 79.5,13.34 79.5,11.05 v79.63,10.92 | U1.14 66.48,10.87 v66.55,10.79
  Bottom 0.254: v66.55,10.79 66.67,10.92 67.69,10.92 67.82,11.05 79.5,11.05 v79.63,10.92
D11_MOSI  (via drill 0.25)
  Top 0.254: U2.MOSI 80.19,11.51 v80.14,11.56 | v67.28,11.56 67.3,11.56 U1.15 67.28,12.61 v66.29,13.59 | JST2.5 66.17,25.79 66.04,25.65 v66.04,24.64 | FLASH.5 85.6,26.67 84.2,28.07 v84.2,28.19 | v77.98,29.08 77.85,28.96 77.09,28.96 76.71,29.34 66.42,29.34 66.17,29.08 65.41,29.08 v65.15,29.34
  Bottom 0.254: v80.14,11.56 v67.28,11.56 | v66.29,13.59 66.17,13.72 66.17,18.8 66.29,18.92 66.29,19.56 65.15,20.7 65.15,24.77 | v84.2,28.19 84.07,28.19 83.06,29.21 78.11,29.21 v77.98,29.08 | 65.15,24.77 v65.15,29.34 | v66.04,24.64 65.28,24.64 65.15,24.77
D12_MISO  (via drill 0.25)
  Top 0.254: v68.07,10.41 U1.16 | U1.16 | U2.MISO 79.7,10.24 v79.63,10.16 | 64.14,25.77 JST2.3 64.16,24.79 v64.14,24.64 | U1.16 68.07,12.7 66.55,14.22 64.14,14.22 v64.01,14.1 | v64.39,29.46 64.39,29.97 64.77,30.35 79.63,30.35 80.77,29.21 FLASH.2
  Bottom 0.254: v68.07,10.41 68.2,10.54 79.12,10.54 79.5,10.16 v79.63,10.16 | v64.01,14.1 64.14,14.22 64.14,17.4 63.88,17.65 63.88,18.16 64.39,18.67 64.39,22.61 64.01,22.99 64.01,24.51 v64.14,24.64 64.01,24.77 64.01,27.05 64.26,27.3 64.26,29.21 v64.39,29.46
D13_SCK  (via drill 0.25)
  Top 0.254: U2.SCK 80.47,12.78 v80.14,12.45 | v69.6,12.57 69.6,13.18 U1.17 68.59,13.2 v67.56,14.22 | v66.93,24.64 67.18,25.77 JST2.6 | FLASH.6 85.34,27.94 84.2,29.08 v84.2,29.72 | v77.34,29.59 77.09,29.84 65.79,29.84 v65.79,29.72
  Bottom 0.254: v80.14,12.45 79.76,12.06 70.1,12.06 v69.6,12.57 | v67.56,14.22 66.67,15.11 66.67,18.54 66.8,18.67 66.8,19.68 65.66,20.83 65.66,23.37 v66.93,24.64 65.66,25.91 65.66,28.96 65.79,29.08 v65.79,29.72 | v84.2,29.72 77.47,29.72 v77.34,29.59
D+
  Top 0.305: U6.4 J5.D+1
D-  (via drill 0.36)
  Top 0.305: J5.D-1 5.61,40.16 v5.97,40.51 | v5.97,38.35 6.62,39.01 U6.5
  Bottom 0.305: v5.97,40.51 5.59,40.13 5.59,38.73 v5.97,38.35
DTR/3  (via drill 0.25)
  Top 0.254: C10.1 13.74,43.46 v13.72,43.43 | U6.28 10.02,43.04 v10.03,43.05
  Bottom 0.254: v10.03,43.05 10.41,43.56 13.59,43.56 v13.72,43.43
GND  (via drill 0.38)
  Top 0.254: U5.ADDR 97.03,28.83 96.9,28.7 96.39,28.7 | C2.2 93.74,23 95.76,25.02 95.76,28.57 95.89,28.7 | U5.GND 96.52,28.83 96.39,28.7 | 96.39,28.7 95.89,28.7 | 95.89,28.7 93.22,28.7 U4.7 U4.GND | U1.21 70.34,16.4 70.61,16.13 71.63,16.13 71.75,16 74.55,16 | 74.55,16 74.55,15.04 C3.1 | 74.55,16 74.55,16.97 C5.2
  Bottom 0.356: BAT1.GND@1 56.66,22.5 57.02,22.86 58.55,22.86 58.93,23.24 58.93,29.08 59.69,29.84 59.82,29.84 v59.94,29.97
  other vias: 88.27,1.02 89.41,1.02 90.55,1.02 60.96,29.97 61.98,29.97 82.55,6.6 81.53,6.6 80.52,6.6 77.85,13.97 77.85,14.99 77.85,16 89.66,28.57 89.66,29.59 89.66,27.56 97.16,21.97 97.16,21.21 78.61,28.07 78.61,27.05 78.61,26.04 67.82,17.34 67.82,16.45 67.82,15.56 69.09,8.13 70.1,8.13 71.12,8.13
  pour Bottom (isolate 0.356): 58.93,32.77 89.92,32.77 89.92,25.02 99.69,25.02 99.69,-0.64 58.93,-0.64
  pour Top (isolate 0.356): 58.93,32.77 89.92,32.77 89.92,25.02 99.69,25.02 99.69,-0.64 58.93,-0.64
GND2  (via drill 0.3)
  Top 0.254: U7.GND 36.96,43.18 36.7,43.43 32.38,43.43 32.13,43.18 U8.GND
  other vias: 33.4,36.83 29.84,36.83
  pour Top (isolate 0.356): 28.07,33.15 40.44,33.15 40.44,44.83 28.07,44.83
  pour Bottom (isolate 0.356): 28.07,33.15 40.44,33.15 40.44,44.83 28.07,44.83
GND3  (via drill 0.25, 0.36)
  Top 0.254: v11.01,39.51 10.51,40.01 U6.3 8.26,40.01 8,40.26 | U6.M 9.41,42.15 9.27,42.29 | LED1.C 20.19,36.48 v20.19,35.81
  Top 0.356: J5.GND1 4.85,38.2 v6.22,36.96
  Bottom 0.254: v20.19,35.81 20.23,35.94
  other vias: 12.7,34.42 11.68,34.42 10.67,34.42 7.11,36.96 4.06,35.43 4.06,36.32 15.49,41.15 15.49,40.26 15.49,39.37 12.03,39.51 11.52,40.01 11.52,39
  pour Top (isolate 0.356): -0.64,33.02 24.44,33.02 24.44,46.35 -0.64,46.35
  pour Bottom (isolate 0.356): -0.64,33.02 24.44,33.02 24.44,46.35 -0.64,46.35
MISO/3  (via drill 0.25)
  Top 0.254: v2.16,44.58 v3.43,44.58
  Bottom 0.254: J6.1 1.79,42.05 2.29,42.55 2.29,44.45 v2.16,44.58 | v3.43,44.58 3.43,44.83 3.68,45.09 17.78,45.09 18.16,44.7 18.16,41.4 18.41,41.15 21.34,41.15 21.84,40.64 21.84,37.47 21.44,37.06 J4.3
MOSI/3
  Bottom 0.254: J6.4 7.04,40.71 6.6,41.15 5.84,41.15 5.59,41.4 5.59,42.8 4.7,43.69 4.7,44.32 4.95,44.58 17.4,44.58 17.65,44.32 17.65,41.15 18.54,40.26 20.21,40.26 J4.5
N$1
  Top 1.27: BAT1.VCC@1 BAT1.GND@2
N$2
  Top 0.254: LED1.A 18.3,34.38 R7.2
N$3
  Top 0.356: J5.VBUS1 3.59,40.8 3.3,40.51 3.3,34.92 3.81,34.42 6.35,34.42 F1.1
N$4
  Bottom 0.356: SJ1.2 11.05,37.08 11.43,37.47 12.45,37.47 12.83,37.08 12.83,36.32 15.49,33.66 20.17,33.66 J4.1
N$5
  Top 0.254: C12.1 R15.1 37.34,37.26 37.34,37.97 37.47,38.1 U7.DVI
N$6
  Top 0.254: LED3.A 18.3,42.26 R8.2
N$7
  Top 0.254: LED2.A 18.3,38.32 R12.2
N$19  (via drill 0.25)
  Top 0.254: R11.1 91.81,23 v91.57,22.99 | v95.63,22.99 95.58,22.99 C23.1 95.59,23.58 97.03,25.02 U5.DVI
  Bottom 0.254: v91.57,22.99 v95.63,22.99
N$29
  Top 0.254: Y1.1 59.8,7.25 59.44,7.62 59.44,13.21 60.23,14 U1.7
N$30
  Top 0.254: Y1.3 60.34,9.26 59.94,9.65 59.94,12.95 60.2,13.21 60.98,13.21 U1.8
N$33
  Top 0.254: U1.20 71.39,15.6 72.01,14.99 72.72,14.99 C3.2
RESET
  Top 0.254: JST2.4 65.16,24.9 64.88,24.62 64.88,22.61 | U1.29 64.88,22.61 | R4.1 61.09,22.61 64.88,22.61
RESET/3  (via drill 0.25)
  Top 0.254: v3.43,43.81 v5.46,43.81 | C10.2 15.54,44.12 v15.41,43.99
  Bottom 0.254: J6.5 2.67,36.97 3.3,37.59 3.3,43.69 v3.43,43.81 | v5.46,43.81 5.71,44.07 15.37,44.07 15.49,43.94 | 15.49,43.94 v15.41,43.99 | v15.41,43.99 15.62,44.07 17.02,44.07 17.14,43.94 17.14,40.89 19.3,38.73 J4.4 | v15.41,43.99 15.41,44.15 15.49,43.94
RX/3  (via drill 0.25)
  Top 0.254: LED2.C 21.24,40.42 21.84,41.02 v21.84,43.18 21.72,43.31 19.43,43.31 19.18,43.56 19.18,44.83 18.92,45.09 17.27,45.09 17.02,44.83 17.02,43.56 16.26,42.8 13.34,42.8 13.21,42.93 11.68,42.93 11.52,42.76 U6.25
  Bottom 0.254: J4.7 21.4,43.62 v21.84,43.18
SCK/3
  Bottom 0.254: J6.3 2.17,39.51 2.79,40.13 2.79,45.09 3.3,45.59 18.03,45.59 18.67,44.96 18.67,42.16 18.92,41.91 20.19,41.91 J4.6
SHIELD_POUR/3
  Top 0.203: J5.SHIELD2 J5.SHIELD3 J5.SHIELD1
TX/3  (via drill 0.25)
  Top 0.254: LED3.C 20.19,44.36 v20.19,44.96 20.19,45.21 19.81,45.59 16.89,45.59 16.51,45.21 16.51,43.94 v16,43.43 | U6.26 11.02,42.89 v10.92,42.93
  Bottom 0.254: v20.19,44.96 20.23,44.83 J4.8 | v10.92,42.93 13.21,42.93 13.34,42.8 14.22,42.8 14.73,43.31 15.88,43.31 v16,43.43
VCC  (via drill 0.25, 0.41)
  Top 0.254: U5.VCC 97.54,30.99 arc90 97.16,31.43 | R5.1 R3.1 | U4.VDD v93.09,26.16 | v93.09,31.11 93.09,31.24 93.22,31.43 | U3.2 75.55,26.43 v75.44,26.42 | v75.44,31.5 75.44,31.43
  Top 0.305: 58.87,14.8 58.8,14.99 | 58.82,16.4 58.8,16.51 | R4.2 58.94,23.63 58.8,23.62 | U2.3.3V 80.57,17.86 | U1.6 68.13,14.8 68.93,14 U1.18 71.09,14 72.14,12.95 72.72,12.95 C4.2 | 80.18,21.2 80.3,21.08 | 86.82,31.32 86.87,31.43 | FLASH.3 83.06,27.94 83.44,28.32 83.44,31.43 | 58.82,25.67 58.8,25.65 | C2.1 93.64,21.04 | 98.17,23.62 98.3,23.5
  Top 0.356: U1.6 58.87,14.8 | U1.4 58.82,16.4 | C1.1 80.3,21.08 80.3,20.07 | 80.3,20.07 80.3,18.13 80.57,17.86 | R3.1 C7.2 80.18,21.2 | 86.82,31.32 FLASH.8 FLASH.7 | 80.3,20.07 85.09,20.07 85.48,20.46 R10.2 R2.2 R1.2 R11.2 C2.1 | JST2.1 58.82,25.67 | 93.64,21.04 94.61,20.07 97.79,20.07 98.3,20.57 98.3,23.5 98.3,30.1 arc90 97.16,31.43 93.22,31.43 86.87,31.43 83.44,31.43 75.44,31.43 59.56,31.43 58.8,30.67 58.8,25.65 58.8,23.62 58.8,16.51 58.8,14.99 58.8,9.14 | S1.P$2 98.17,23.62 | BAT1.VCC@2 56,9.4 56.26,9.14 58.8,9.14 | 58.8,9.14 58.8,5.59 59.2,5.19 J1.4 63.14,3.54 63.5,3.17 v66.42,3.17 | J3.4 83.58,5.19 v83.57,5.21 | J2.4 73.39,5.19 v73.15,5.21
  Bottom 0.254: v93.09,26.16 v93.09,31.11 | v75.44,26.42 v75.44,31.5
  Bottom 0.356: v83.57,5.21 v73.15,5.21 69.85,5.21 69.72,5.08 BAT2.+ 69.15,3.17 v66.42,3.17
VCC/2  (via drill 0.3)
  Top 0.254: U8.VDD 32.13,39.24 32,39.12 32,38.61 | 32,38.61 32,36.96 | 32,36.96 32,36.2 J7.4 | C11.1 31.91,36.87 32,36.96 | R15.2 38.75,41.8 U7.VCC 37.97,41.15 37.85,41.02 36.07,41.02 35.05,40.01 34.29,40.01 v34.16,40.13 | v34.16,38.86 33.91,38.61 32,38.61
  Bottom 0.254: v34.16,40.13 v34.16,38.86

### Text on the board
tPlace: SENSOR BOARD
bPlace: TX | RX | SCK | MOSI | RST | -5V | 3.3V | MISO | 3.3V | SDA | SCL | GND | GND | VCC | 2018/03 | V1.0
Document: GREEN | YELLOW | BLUE | ORANGE | WHITE | VIOLET | BLACK | RED

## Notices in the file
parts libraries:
SparkFun-DigitalIC: Licensing: Creative Commons ShareAlike 4.0 International - https://creativecommons.org/licenses/by-sa/4.0
SparkFun-Aesthetics: Licensing: CC v3.0 Share-Alike You are welcome to use this library for commercial purposes.
